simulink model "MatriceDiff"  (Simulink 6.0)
settings: Solver=ode45  StartTime=0  StopTime=17*t0  RelTol=1e-3
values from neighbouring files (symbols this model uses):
  b = S/Sm    (= 0.1)    [Constantes.m]    (also in ConstantesBck.m)
  beta = 0.95    [Constantes.m]    (also in ConstantesBck.m; ResCourV1.m = 1; ResCrV1.m = 1; ResEnerV1.m = 1)
  C = 1    [Constantes.m]    (also in ConstantesBck.m)
  gk = 36    [Constantes.m]    (also in ConstantesBck.m; sim_hh.m)
  gl = 0.3    [Constantes.m]    (also in ConstantesBck.m; sim_hh.m)
  gna = 120    [Constantes.m]    (also in ConstantesBck.m; sim_hh.m)
  h0 = 0.5961    [Constantes.m]    (also in ConstantesBck.m)
  m0 = 0.0529    [Constantes.m]    (also in ConstantesBck.m)
  mK = 0    [Constantes.m]    (also in ConstantesBck.m)
  mL = 0    [Constantes.m]    (also in ConstantesBck.m)
  mNa = 0    [Constantes.m]    (also in ConstantesBck.m)
  N = [6,8,5,5,7,1,2,6,9,1,1,9,4,8,8,7]    [Constantes.m]    (also in ConstantesBck.m; ImpedanceZtissus.m = 100; Ztissus.m = 100; charge.m = N(:,2))
  n0 = 0.3177    [Constantes.m]    (also in ConstantesBck.m)
  rapportIE = 10    [Constantes.m]
  Sm = 3.14e-2    (= 0.0314)    [Constantes.m]    (also in ConstantesBck.m = 0.000314)
  t0 = 2E-3    (= 0.002)    [Constantes.m]    (also in ConstantesBck.m = 0.001)
  Vk = -82    [Constantes.m]    (also in ConstantesBck.m)
  Vl = -59    [Constantes.m]    (also in ConstantesBck.m)
  Vna = 45    [Constantes.m]    (also in ConstantesBck.m)
  Vr = -70    [Constantes.m]    (also in ConstantesBck.m)
undefined symbols (not defined in the file or in its folder): ln
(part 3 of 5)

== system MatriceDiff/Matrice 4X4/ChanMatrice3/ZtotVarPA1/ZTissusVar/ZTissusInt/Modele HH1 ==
  HHin : Inport  Port=1  LatchInput=off
  VRefIn : Inport  Port=2  LatchInput=off
  FK : Subsystem
  FL : Fcn  Expr=gl*(u-Vl)
  FNa : Subsystem
  Gain : Gain  Gain=(1-b)/C
  Gain1 : Gain  Gain=1/(Sm*(1-b))
  Gain2 : Gain  Gain=1+mK*(b/(1-b))
  Gain3 : Gain  Gain=1+mL*(b/(1-b))
  Gain4 : Gain  Gain=1+mNa*(b/(1-b))
  Integrator : Integrator  InitialCondition=Vr
  Sum : Sum  Inputs=|---+
  Sum1 : Sum  Inputs=|++
  HHout : Outport
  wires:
  Sum/1 -> Gain/1
  Gain/1 -> Integrator/1
  FK/1(FKout) -> Gain4/1
  FNa/1(FNaOut) -> Gain2/1
  FL/1 -> Gain3/1
  HHin/1 -> Gain1/1
  Integrator/1 -> Sum1/1
  Sum1/1 -> HHout/1, FNa/1(FNaIn), FL/1, FK/1(FKIn)
  VRefIn/1 -> Sum1/2
  Gain1/1 -> Sum/4
  Gain4/1 -> Sum/1
  Gain2/1 -> Sum/2
  Gain3/1 -> Sum/3

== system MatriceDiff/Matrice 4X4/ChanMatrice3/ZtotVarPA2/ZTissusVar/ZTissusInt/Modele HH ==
  HHin : Inport  Port=1  LatchInput=off
  VRefIn : Inport  Port=2  LatchInput=off
  FK : Subsystem
  FL : Fcn  Expr=gl*(u-Vl)
  FNa : Subsystem
  Gain : Gain  Gain=(1-b)/C
  Gain1 : Gain  Gain=1/(Sm*(1-b))
  Gain2 : Gain  Gain=1+mK*(b/(1-b))
  Gain3 : Gain  Gain=1+mL*(b/(1-b))
  Gain4 : Gain  Gain=1+mNa*(b/(1-b))
  Integrator : Integrator  InitialCondition=Vr
  Sum : Sum  Inputs=|---+
  Sum1 : Sum  Inputs=|+-
  HHout : Outport
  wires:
  Sum/1 -> Gain/1
  Gain/1 -> Integrator/1
  FK/1(FKout) -> Gain4/1
  FNa/1(FNaOut) -> Gain2/1
  FL/1 -> Gain3/1
  HHin/1 -> Gain1/1
  Integrator/1 -> Sum1/1
  Sum1/1 -> HHout/1, FNa/1(FNaIn), FL/1, FK/1(FKIn)
  VRefIn/1 -> Sum1/2
  Gain1/1 -> Sum/4
  Gain4/1 -> Sum/1
  Gain2/1 -> Sum/2
  Gain3/1 -> Sum/3

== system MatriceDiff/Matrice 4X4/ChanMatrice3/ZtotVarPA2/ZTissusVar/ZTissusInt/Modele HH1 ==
  HHin : Inport  Port=1  LatchInput=off
  VRefIn : Inport  Port=2  LatchInput=off
  FK : Subsystem
  FL : Fcn  Expr=gl*(u-Vl)
  FNa : Subsystem
  Gain : Gain  Gain=(1-b)/C
  Gain1 : Gain  Gain=1/(Sm*(1-b))
  Gain2 : Gain  Gain=1+mK*(b/(1-b))
  Gain3 : Gain  Gain=1+mL*(b/(1-b))
  Gain4 : Gain  Gain=1+mNa*(b/(1-b))
  Integrator : Integrator  InitialCondition=Vr
  Sum : Sum  Inputs=|---+
  Sum1 : Sum  Inputs=|++
  HHout : Outport
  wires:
  Sum/1 -> Gain/1
  Gain/1 -> Integrator/1
  FK/1(FKout) -> Gain4/1
  FNa/1(FNaOut) -> Gain2/1
  FL/1 -> Gain3/1
  HHin/1 -> Gain1/1
  Integrator/1 -> Sum1/1
  Sum1/1 -> HHout/1, FNa/1(FNaIn), FL/1, FK/1(FKIn)
  VRefIn/1 -> Sum1/2
  Gain1/1 -> Sum/4
  Gain4/1 -> Sum/1
  Gain2/1 -> Sum/2
  Gain3/1 -> Sum/3

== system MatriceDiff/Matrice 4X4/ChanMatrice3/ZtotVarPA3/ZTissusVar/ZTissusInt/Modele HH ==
  HHin : Inport  Port=1  LatchInput=off
  VRefIn : Inport  Port=2  LatchInput=off
  FK : Subsystem
  FL : Fcn  Expr=gl*(u-Vl)
  FNa : Subsystem
  Gain : Gain  Gain=(1-b)/C
  Gain1 : Gain  Gain=1/(Sm*(1-b))
  Gain2 : Gain  Gain=1+mK*(b/(1-b))
  Gain3 : Gain  Gain=1+mL*(b/(1-b))
  Gain4 : Gain  Gain=1+mNa*(b/(1-b))
  Integrator : Integrator  InitialCondition=Vr
  Sum : Sum  Inputs=|---+
  Sum1 : Sum  Inputs=|+-
  HHout : Outport
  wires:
  Sum/1 -> Gain/1
  Gain/1 -> Integrator/1
  FK/1(FKout) -> Gain4/1
  FNa/1(FNaOut) -> Gain2/1
  FL/1 -> Gain3/1
  HHin/1 -> Gain1/1
  Integrator/1 -> Sum1/1
  Sum1/1 -> HHout/1, FNa/1(FNaIn), FL/1, FK/1(FKIn)
  VRefIn/1 -> Sum1/2
  Gain1/1 -> Sum/4
  Gain4/1 -> Sum/1
  Gain2/1 -> Sum/2
  Gain3/1 -> Sum/3

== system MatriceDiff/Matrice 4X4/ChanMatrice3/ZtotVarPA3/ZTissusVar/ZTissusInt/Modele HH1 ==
  HHin : Inport  Port=1  LatchInput=off
  VRefIn : Inport  Port=2  LatchInput=off
  FK : Subsystem
  FL : Fcn  Expr=gl*(u-Vl)
  FNa : Subsystem
  Gain : Gain  Gain=(1-b)/C
  Gain1 : Gain  Gain=1/(Sm*(1-b))
  Gain2 : Gain  Gain=1+mK*(b/(1-b))
  Gain3 : Gain  Gain=1+mL*(b/(1-b))
  Gain4 : Gain  Gain=1+mNa*(b/(1-b))
  Integrator : Integrator  InitialCondition=Vr
  Sum : Sum  Inputs=|---+
  Sum1 : Sum  Inputs=|++
  HHout : Outport
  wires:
  Sum/1 -> Gain/1
  Gain/1 -> Integrator/1
  FK/1(FKout) -> Gain4/1
  FNa/1(FNaOut) -> Gain2/1
  FL/1 -> Gain3/1
  HHin/1 -> Gain1/1
  Integrator/1 -> Sum1/1
  Sum1/1 -> HHout/1, FNa/1(FNaIn), FL/1, FK/1(FKIn)
  VRefIn/1 -> Sum1/2
  Gain1/1 -> Sum/4
  Gain4/1 -> Sum/1
  Gain2/1 -> Sum/2
  Gain3/1 -> Sum/3

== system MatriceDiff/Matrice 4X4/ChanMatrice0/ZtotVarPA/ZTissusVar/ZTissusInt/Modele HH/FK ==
  note: gkm
  note: (Vm-Vk0)
  FKIn : Inport  Port=1  LatchInput=off
  (Vm-Vk0) : Fcn  Expr=(u-Vk)
  Product : Product
  n(Vm) : Subsystem
  n^4 : Fcn  Expr=gk*(u^4)
  FKout : Outport  InitialOutput=0
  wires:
  n(Vm)/1(n) -> n^4/1
  (Vm-Vk0)/1 -> Product/2
  Product/1 -> FKout/1
  n^4/1 -> Product/1
  FKIn/1 -> n(Vm)/1(Vm), (Vm-Vk0)/1

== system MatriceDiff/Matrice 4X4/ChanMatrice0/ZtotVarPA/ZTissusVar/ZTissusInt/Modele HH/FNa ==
  note: gNa*m^3
  note: m
  note: h
  note: gNam
  note: (Vm-VNa0)
  FNaIn : Inport  Port=1  LatchInput=off
  (Vm-VNa0) : Fcn  Expr=(u-Vna)
  Product : Product
  Product1 : Product
  gna*m^3 : Fcn  Expr=gna*u^3
  h(Vm) : Subsystem
  m(Vm) : Subsystem
  FNaOut : Outport  InitialOutput=0
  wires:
  (Vm-VNa0)/1 -> Product1/2
  gna*m^3/1 -> Product/1
  Product1/1 -> FNaOut/1
  FNaIn/1 -> m(Vm)/1(Vm), h(Vm)/1(Vm), (Vm-VNa0)/1
  m(Vm)/1(n) -> gna*m^3/1
  h(Vm)/1(h) -> Product/2
  Product/1 -> Product1/1

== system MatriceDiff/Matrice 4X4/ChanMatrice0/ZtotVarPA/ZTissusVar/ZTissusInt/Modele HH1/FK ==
  note: gkm
  note: (Vm-Vk0)
  FKIn : Inport  Port=1  LatchInput=off
  (Vm-Vk0) : Fcn  Expr=(u-Vk)
  Product : Product
  n(Vm) : Subsystem
  n^4 : Fcn  Expr=gk*(u^4)
  FKout : Outport  InitialOutput=0
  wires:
  n(Vm)/1(n) -> n^4/1
  (Vm-Vk0)/1 -> Product/2
  Product/1 -> FKout/1
  n^4/1 -> Product/1
  FKIn/1 -> n(Vm)/1(Vm), (Vm-Vk0)/1

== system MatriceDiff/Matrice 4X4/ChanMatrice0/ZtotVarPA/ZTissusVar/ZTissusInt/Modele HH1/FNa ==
  note: gNa*m^3
  note: m
  note: h
  note: gNam
  note: (Vm-VNa0)
  FNaIn : Inport  Port=1  LatchInput=off
  (Vm-VNa0) : Fcn  Expr=(u-Vna)
  Product : Product
  Product1 : Product
  gna*m^3 : Fcn  Expr=gna*u^3
  h(Vm) : Subsystem
  m(Vm) : Subsystem
  FNaOut : Outport  InitialOutput=0
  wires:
  (Vm-VNa0)/1 -> Product1/2
  gna*m^3/1 -> Product/1
  Product1/1 -> FNaOut/1
  FNaIn/1 -> m(Vm)/1(Vm), h(Vm)/1(Vm), (Vm-VNa0)/1
  m(Vm)/1(n) -> gna*m^3/1
  h(Vm)/1(h) -> Product/2
  Product/1 -> Product1/1

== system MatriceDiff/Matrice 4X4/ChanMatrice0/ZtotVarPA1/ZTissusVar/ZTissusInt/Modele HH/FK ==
  note: gkm
  note: (Vm-Vk0)
  FKIn : Inport  Port=1  LatchInput=off
  (Vm-Vk0) : Fcn  Expr=(u-Vk)
  Product : Product
  n(Vm) : Subsystem
  n^4 : Fcn  Expr=gk*(u^4)
  FKout : Outport  InitialOutput=0
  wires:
  n(Vm)/1(n) -> n^4/1
  (Vm-Vk0)/1 -> Product/2
  Product/1 -> FKout/1
  n^4/1 -> Product/1
  FKIn/1 -> n(Vm)/1(Vm), (Vm-Vk0)/1

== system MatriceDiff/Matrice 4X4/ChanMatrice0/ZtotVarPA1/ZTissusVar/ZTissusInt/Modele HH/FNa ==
  note: gNa*m^3
  note: m
  note: h
  note: gNam
  note: (Vm-VNa0)
  FNaIn : Inport  Port=1  LatchInput=off
  (Vm-VNa0) : Fcn  Expr=(u-Vna)
  Product : Product
  Product1 : Product
  gna*m^3 : Fcn  Expr=gna*u^3
  h(Vm) : Subsystem
  m(Vm) : Subsystem
  FNaOut : Outport  InitialOutput=0
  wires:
  (Vm-VNa0)/1 -> Product1/2
  gna*m^3/1 -> Product/1
  Product1/1 -> FNaOut/1
  FNaIn/1 -> m(Vm)/1(Vm), h(Vm)/1(Vm), (Vm-VNa0)/1
  m(Vm)/1(n) -> gna*m^3/1
  h(Vm)/1(h) -> Product/2
  Product/1 -> Product1/1

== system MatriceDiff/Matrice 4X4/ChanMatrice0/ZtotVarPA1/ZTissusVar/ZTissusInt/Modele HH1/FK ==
  note: gkm
  note: (Vm-Vk0)
  FKIn : Inport  Port=1  LatchInput=off
  (Vm-Vk0) : Fcn  Expr=(u-Vk)
  Product : Product
  n(Vm) : Subsystem
  n^4 : Fcn  Expr=gk*(u^4)
  FKout : Outport  InitialOutput=0
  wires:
  n(Vm)/1(n) -> n^4/1
  (Vm-Vk0)/1 -> Product/2
  Product/1 -> FKout/1
  n^4/1 -> Product/1
  FKIn/1 -> n(Vm)/1(Vm), (Vm-Vk0)/1

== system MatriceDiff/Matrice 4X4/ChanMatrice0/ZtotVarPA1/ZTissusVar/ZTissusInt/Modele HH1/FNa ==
  note: gNa*m^3
  note: m
  note: h
  note: gNam
  note: (Vm-VNa0)
  FNaIn : Inport  Port=1  LatchInput=off
  (Vm-VNa0) : Fcn  Expr=(u-Vna)
  Product : Product
  Product1 : Product
  gna*m^3 : Fcn  Expr=gna*u^3
  h(Vm) : Subsystem
  m(Vm) : Subsystem
  FNaOut : Outport  InitialOutput=0
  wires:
  (Vm-VNa0)/1 -> Product1/2
  gna*m^3/1 -> Product/1
  Product1/1 -> FNaOut/1
  FNaIn/1 -> m(Vm)/1(Vm), h(Vm)/1(Vm), (Vm-VNa0)/1
  m(Vm)/1(n) -> gna*m^3/1
  h(Vm)/1(h) -> Product/2
  Product/1 -> Product1/1

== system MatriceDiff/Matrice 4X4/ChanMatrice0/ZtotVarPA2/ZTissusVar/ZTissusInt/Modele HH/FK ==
  note: gkm
  note: (Vm-Vk0)
  FKIn : Inport  Port=1  LatchInput=off
  (Vm-Vk0) : Fcn  Expr=(u-Vk)
  Product : Product
  n(Vm) : Subsystem
  n^4 : Fcn  Expr=gk*(u^4)
  FKout : Outport  InitialOutput=0
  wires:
  n(Vm)/1(n) -> n^4/1
  (Vm-Vk0)/1 -> Product/2
  Product/1 -> FKout/1
  n^4/1 -> Product/1
  FKIn/1 -> n(Vm)/1(Vm), (Vm-Vk0)/1

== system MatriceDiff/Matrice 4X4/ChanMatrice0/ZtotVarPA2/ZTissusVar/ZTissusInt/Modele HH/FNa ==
  note: gNa*m^3
  note: m
  note: h
  note: gNam
  note: (Vm-VNa0)
  FNaIn : Inport  Port=1  LatchInput=off
  (Vm-VNa0) : Fcn  Expr=(u-Vna)
  Product : Product
  Product1 : Product
  gna*m^3 : Fcn  Expr=gna*u^3
  h(Vm) : Subsystem
  m(Vm) : Subsystem
  FNaOut : Outport  InitialOutput=0
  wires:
  (Vm-VNa0)/1 -> Product1/2
  gna*m^3/1 -> Product/1
  Product1/1 -> FNaOut/1
  FNaIn/1 -> m(Vm)/1(Vm), h(Vm)/1(Vm), (Vm-VNa0)/1
  m(Vm)/1(n) -> gna*m^3/1
  h(Vm)/1(h) -> Product/2
  Product/1 -> Product1/1

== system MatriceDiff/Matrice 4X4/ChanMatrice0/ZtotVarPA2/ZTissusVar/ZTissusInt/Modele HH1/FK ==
  note: gkm
  note: (Vm-Vk0)
  FKIn : Inport  Port=1  LatchInput=off
  (Vm-Vk0) : Fcn  Expr=(u-Vk)
  Product : Product
  n(Vm) : Subsystem
  n^4 : Fcn  Expr=gk*(u^4)
  FKout : Outport  InitialOutput=0
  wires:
  n(Vm)/1(n) -> n^4/1
  (Vm-Vk0)/1 -> Product/2
  Product/1 -> FKout/1
  n^4/1 -> Product/1
  FKIn/1 -> n(Vm)/1(Vm), (Vm-Vk0)/1

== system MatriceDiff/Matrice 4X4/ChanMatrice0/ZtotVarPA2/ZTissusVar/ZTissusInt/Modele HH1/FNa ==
  note: gNa*m^3
  note: m
  note: h
  note: gNam
  note: (Vm-VNa0)
  FNaIn : Inport  Port=1  LatchInput=off
  (Vm-VNa0) : Fcn  Expr=(u-Vna)
  Product : Product
  Product1 : Product
  gna*m^3 : Fcn  Expr=gna*u^3
  h(Vm) : Subsystem
  m(Vm) : Subsystem
  FNaOut : Outport  InitialOutput=0
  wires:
  (Vm-VNa0)/1 -> Product1/2
  gna*m^3/1 -> Product/1
  Product1/1 -> FNaOut/1
  FNaIn/1 -> m(Vm)/1(Vm), h(Vm)/1(Vm), (Vm-VNa0)/1
  m(Vm)/1(n) -> gna*m^3/1
  h(Vm)/1(h) -> Product/2
  Product/1 -> Product1/1

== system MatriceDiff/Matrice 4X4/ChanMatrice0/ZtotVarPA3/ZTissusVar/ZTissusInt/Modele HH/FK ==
  note: gkm
  note: (Vm-Vk0)
  FKIn : Inport  Port=1  LatchInput=off
  (Vm-Vk0) : Fcn  Expr=(u-Vk)
  Product : Product
  n(Vm) : Subsystem
  n^4 : Fcn  Expr=gk*(u^4)
  FKout : Outport  InitialOutput=0
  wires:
  n(Vm)/1(n) -> n^4/1
  (Vm-Vk0)/1 -> Product/2
  Product/1 -> FKout/1
  n^4/1 -> Product/1
  FKIn/1 -> n(Vm)/1(Vm), (Vm-Vk0)/1

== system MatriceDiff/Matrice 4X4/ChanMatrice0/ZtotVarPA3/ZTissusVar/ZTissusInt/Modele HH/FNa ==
  note: gNa*m^3
  note: m
  note: h
  note: gNam
  note: (Vm-VNa0)
  FNaIn : Inport  Port=1  LatchInput=off
  (Vm-VNa0) : Fcn  Expr=(u-Vna)
  Product : Product
  Product1 : Product
  gna*m^3 : Fcn  Expr=gna*u^3
  h(Vm) : Subsystem
  m(Vm) : Subsystem
  FNaOut : Outport  InitialOutput=0
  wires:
  (Vm-VNa0)/1 -> Product1/2
  gna*m^3/1 -> Product/1
  Product1/1 -> FNaOut/1
  FNaIn/1 -> m(Vm)/1(Vm), h(Vm)/1(Vm), (Vm-VNa0)/1
  m(Vm)/1(n) -> gna*m^3/1
  h(Vm)/1(h) -> Product/2
  Product/1 -> Product1/1

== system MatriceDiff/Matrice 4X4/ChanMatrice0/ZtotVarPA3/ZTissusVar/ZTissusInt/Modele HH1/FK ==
  note: gkm
  note: (Vm-Vk0)
  FKIn : Inport  Port=1  LatchInput=off
  (Vm-Vk0) : Fcn  Expr=(u-Vk)
  Product : Product
  n(Vm) : Subsystem
  n^4 : Fcn  Expr=gk*(u^4)
  FKout : Outport  InitialOutput=0
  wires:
  n(Vm)/1(n) -> n^4/1
  (Vm-Vk0)/1 -> Product/2
  Product/1 -> FKout/1
  n^4/1 -> Product/1
  FKIn/1 -> n(Vm)/1(Vm), (Vm-Vk0)/1

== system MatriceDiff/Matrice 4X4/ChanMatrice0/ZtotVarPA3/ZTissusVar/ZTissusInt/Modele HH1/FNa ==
  note: gNa*m^3
  note: m
  note: h
  note: gNam
  note: (Vm-VNa0)
  FNaIn : Inport  Port=1  LatchInput=off
  (Vm-VNa0) : Fcn  Expr=(u-Vna)
  Product : Product
  Product1 : Product
  gna*m^3 : Fcn  Expr=gna*u^3
  h(Vm) : Subsystem
  m(Vm) : Subsystem
  FNaOut : Outport  InitialOutput=0
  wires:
  (Vm-VNa0)/1 -> Product1/2
  gna*m^3/1 -> Product/1
  Product1/1 -> FNaOut/1
  FNaIn/1 -> m(Vm)/1(Vm), h(Vm)/1(Vm), (Vm-VNa0)/1
  m(Vm)/1(n) -> gna*m^3/1
  h(Vm)/1(h) -> Product/2
  Product/1 -> Product1/1

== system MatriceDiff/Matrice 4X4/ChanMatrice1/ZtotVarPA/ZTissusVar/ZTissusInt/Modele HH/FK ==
  note: gkm
  note: (Vm-Vk0)
  FKIn : Inport  Port=1  LatchInput=off
  (Vm-Vk0) : Fcn  Expr=(u-Vk)
  Product : Product
  n(Vm) : Subsystem
  n^4 : Fcn  Expr=gk*(u^4)
  FKout : Outport  InitialOutput=0
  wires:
  n(Vm)/1(n) -> n^4/1
  (Vm-Vk0)/1 -> Product/2
  Product/1 -> FKout/1
  n^4/1 -> Product/1
  FKIn/1 -> n(Vm)/1(Vm), (Vm-Vk0)/1

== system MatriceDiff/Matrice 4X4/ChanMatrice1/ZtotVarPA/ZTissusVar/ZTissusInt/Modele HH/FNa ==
  note: gNa*m^3
  note: m
  note: h
  note: gNam
  note: (Vm-VNa0)
  FNaIn : Inport  Port=1  LatchInput=off
  (Vm-VNa0) : Fcn  Expr=(u-Vna)
  Product : Product
  Product1 : Product
  gna*m^3 : Fcn  Expr=gna*u^3
  h(Vm) : Subsystem
  m(Vm) : Subsystem
  FNaOut : Outport  InitialOutput=0
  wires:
  (Vm-VNa0)/1 -> Product1/2
  gna*m^3/1 -> Product/1
  Product1/1 -> FNaOut/1
  FNaIn/1 -> m(Vm)/1(Vm), h(Vm)/1(Vm), (Vm-VNa0)/1
  m(Vm)/1(n) -> gna*m^3/1
  h(Vm)/1(h) -> Product/2
  Product/1 -> Product1/1

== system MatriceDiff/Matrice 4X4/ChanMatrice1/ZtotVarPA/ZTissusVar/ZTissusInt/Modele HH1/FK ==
  note: gkm
  note: (Vm-Vk0)
  FKIn : Inport  Port=1  LatchInput=off
  (Vm-Vk0) : Fcn  Expr=(u-Vk)
  Product : Product
  n(Vm) : Subsystem
  n^4 : Fcn  Expr=gk*(u^4)
  FKout : Outport  InitialOutput=0
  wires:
  n(Vm)/1(n) -> n^4/1
  (Vm-Vk0)/1 -> Product/2
  Product/1 -> FKout/1
  n^4/1 -> Product/1
  FKIn/1 -> n(Vm)/1(Vm), (Vm-Vk0)/1

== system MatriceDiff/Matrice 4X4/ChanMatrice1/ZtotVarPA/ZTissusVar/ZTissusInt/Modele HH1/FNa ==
  note: gNa*m^3
  note: m
  note: h
  note: gNam
  note: (Vm-VNa0)
  FNaIn : Inport  Port=1  LatchInput=off
  (Vm-VNa0) : Fcn  Expr=(u-Vna)
  Product : Product
  Product1 : Product
  gna*m^3 : Fcn  Expr=gna*u^3
  h(Vm) : Subsystem
  m(Vm) : Subsystem
  FNaOut : Outport  InitialOutput=0
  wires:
  (Vm-VNa0)/1 -> Product1/2
  gna*m^3/1 -> Product/1
  Product1/1 -> FNaOut/1
  FNaIn/1 -> m(Vm)/1(Vm), h(Vm)/1(Vm), (Vm-VNa0)/1
  m(Vm)/1(n) -> gna*m^3/1
  h(Vm)/1(h) -> Product/2
  Product/1 -> Product1/1

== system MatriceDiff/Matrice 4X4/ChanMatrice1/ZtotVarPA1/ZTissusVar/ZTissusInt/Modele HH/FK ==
  note: gkm
  note: (Vm-Vk0)
  FKIn : Inport  Port=1  LatchInput=off
  (Vm-Vk0) : Fcn  Expr=(u-Vk)
  Product : Product
  n(Vm) : Subsystem
  n^4 : Fcn  Expr=gk*(u^4)
  FKout : Outport  InitialOutput=0
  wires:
  n(Vm)/1(n) -> n^4/1
  (Vm-Vk0)/1 -> Product/2
  Product/1 -> FKout/1
  n^4/1 -> Product/1
  FKIn/1 -> n(Vm)/1(Vm), (Vm-Vk0)/1

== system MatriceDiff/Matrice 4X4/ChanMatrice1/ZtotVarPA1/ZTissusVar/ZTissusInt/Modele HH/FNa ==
  note: gNa*m^3
  note: m
  note: h
  note: gNam
  note: (Vm-VNa0)
  FNaIn : Inport  Port=1  LatchInput=off
  (Vm-VNa0) : Fcn  Expr=(u-Vna)
  Product : Product
  Product1 : Product
  gna*m^3 : Fcn  Expr=gna*u^3
  h(Vm) : Subsystem
  m(Vm) : Subsystem
  FNaOut : Outport  InitialOutput=0
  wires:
  (Vm-VNa0)/1 -> Product1/2
  gna*m^3/1 -> Product/1
  Product1/1 -> FNaOut/1
  FNaIn/1 -> m(Vm)/1(Vm), h(Vm)/1(Vm), (Vm-VNa0)/1
  m(Vm)/1(n) -> gna*m^3/1
  h(Vm)/1(h) -> Product/2
  Product/1 -> Product1/1

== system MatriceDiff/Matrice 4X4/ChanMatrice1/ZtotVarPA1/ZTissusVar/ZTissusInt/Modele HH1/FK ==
  note: gkm
  note: (Vm-Vk0)
  FKIn : Inport  Port=1  LatchInput=off
  (Vm-Vk0) : Fcn  Expr=(u-Vk)
  Product : Product
  n(Vm) : Subsystem
  n^4 : Fcn  Expr=gk*(u^4)
  FKout : Outport  InitialOutput=0
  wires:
  n(Vm)/1(n) -> n^4/1
  (Vm-Vk0)/1 -> Product/2
  Product/1 -> FKout/1
  n^4/1 -> Product/1
  FKIn/1 -> n(Vm)/1(Vm), (Vm-Vk0)/1

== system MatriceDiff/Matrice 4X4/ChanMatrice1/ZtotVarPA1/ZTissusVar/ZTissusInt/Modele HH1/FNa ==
  note: gNa*m^3
  note: m
  note: h
  note: gNam
  note: (Vm-VNa0)
  FNaIn : Inport  Port=1  LatchInput=off
  (Vm-VNa0) : Fcn  Expr=(u-Vna)
  Product : Product
  Product1 : Product
  gna*m^3 : Fcn  Expr=gna*u^3
  h(Vm) : Subsystem
  m(Vm) : Subsystem
  FNaOut : Outport  InitialOutput=0
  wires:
  (Vm-VNa0)/1 -> Product1/2
  gna*m^3/1 -> Product/1
  Product1/1 -> FNaOut/1
  FNaIn/1 -> m(Vm)/1(Vm), h(Vm)/1(Vm), (Vm-VNa0)/1
  m(Vm)/1(n) -> gna*m^3/1
  h(Vm)/1(h) -> Product/2
  Product/1 -> Product1/1

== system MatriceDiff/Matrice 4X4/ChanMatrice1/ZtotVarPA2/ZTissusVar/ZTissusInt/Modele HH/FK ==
  note: gkm
  note: (Vm-Vk0)
  FKIn : Inport  Port=1  LatchInput=off
  (Vm-Vk0) : Fcn  Expr=(u-Vk)
  Product : Product
  n(Vm) : Subsystem
  n^4 : Fcn  Expr=gk*(u^4)
  FKout : Outport  InitialOutput=0
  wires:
  n(Vm)/1(n) -> n^4/1
  (Vm-Vk0)/1 -> Product/2
  Product/1 -> FKout/1
  n^4/1 -> Product/1
  FKIn/1 -> n(Vm)/1(Vm), (Vm-Vk0)/1

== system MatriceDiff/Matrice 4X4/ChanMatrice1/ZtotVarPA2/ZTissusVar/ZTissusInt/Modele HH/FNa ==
  note: gNa*m^3
  note: m
  note: h
  note: gNam
  note: (Vm-VNa0)
  FNaIn : Inport  Port=1  LatchInput=off
  (Vm-VNa0) : Fcn  Expr=(u-Vna)
  Product : Product
  Product1 : Product
  gna*m^3 : Fcn  Expr=gna*u^3
  h(Vm) : Subsystem
  m(Vm) : Subsystem
  FNaOut : Outport  InitialOutput=0
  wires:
  (Vm-VNa0)/1 -> Product1/2
  gna*m^3/1 -> Product/1
  Product1/1 -> FNaOut/1
  FNaIn/1 -> m(Vm)/1(Vm), h(Vm)/1(Vm), (Vm-VNa0)/1
  m(Vm)/1(n) -> gna*m^3/1
  h(Vm)/1(h) -> Product/2
  Product/1 -> Product1/1

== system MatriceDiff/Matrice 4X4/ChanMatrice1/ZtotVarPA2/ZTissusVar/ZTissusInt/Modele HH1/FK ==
  note: gkm
  note: (Vm-Vk0)
  FKIn : Inport  Port=1  LatchInput=off
  (Vm-Vk0) : Fcn  Expr=(u-Vk)
  Product : Product
  n(Vm) : Subsystem
  n^4 : Fcn  Expr=gk*(u^4)
  FKout : Outport  InitialOutput=0
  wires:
  n(Vm)/1(n) -> n^4/1
  (Vm-Vk0)/1 -> Product/2
  Product/1 -> FKout/1
  n^4/1 -> Product/1
  FKIn/1 -> n(Vm)/1(Vm), (Vm-Vk0)/1

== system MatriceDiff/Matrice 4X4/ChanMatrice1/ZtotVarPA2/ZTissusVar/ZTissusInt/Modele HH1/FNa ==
  note: gNa*m^3
  note: m
  note: h
  note: gNam
  note: (Vm-VNa0)
  FNaIn : Inport  Port=1  LatchInput=off
  (Vm-VNa0) : Fcn  Expr=(u-Vna)
  Product : Product
  Product1 : Product
  gna*m^3 : Fcn  Expr=gna*u^3
  h(Vm) : Subsystem
  m(Vm) : Subsystem
  FNaOut : Outport  InitialOutput=0
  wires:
  (Vm-VNa0)/1 -> Product1/2
  gna*m^3/1 -> Product/1
  Product1/1 -> FNaOut/1
  FNaIn/1 -> m(Vm)/1(Vm), h(Vm)/1(Vm), (Vm-VNa0)/1
  m(Vm)/1(n) -> gna*m^3/1
  h(Vm)/1(h) -> Product/2
  Product/1 -> Product1/1

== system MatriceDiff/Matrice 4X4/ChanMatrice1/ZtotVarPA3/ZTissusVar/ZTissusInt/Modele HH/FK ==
  note: gkm
  note: (Vm-Vk0)
  FKIn : Inport  Port=1  LatchInput=off
  (Vm-Vk0) : Fcn  Expr=(u-Vk)
  Product : Product
  n(Vm) : Subsystem
  n^4 : Fcn  Expr=gk*(u^4)
  FKout : Outport  InitialOutput=0
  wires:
  n(Vm)/1(n) -> n^4/1
  (Vm-Vk0)/1 -> Product/2
  Product/1 -> FKout/1
  n^4/1 -> Product/1
  FKIn/1 -> n(Vm)/1(Vm), (Vm-Vk0)/1

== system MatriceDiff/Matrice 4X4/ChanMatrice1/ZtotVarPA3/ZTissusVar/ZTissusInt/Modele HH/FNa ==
  note: gNa*m^3
  note: m
  note: h
  note: gNam
  note: (Vm-VNa0)
  FNaIn : Inport  Port=1  LatchInput=off
  (Vm-VNa0) : Fcn  Expr=(u-Vna)
  Product : Product
  Product1 : Product
  gna*m^3 : Fcn  Expr=gna*u^3
  h(Vm) : Subsystem
  m(Vm) : Subsystem
  FNaOut : Outport  InitialOutput=0
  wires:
  (Vm-VNa0)/1 -> Product1/2
  gna*m^3/1 -> Product/1
  Product1/1 -> FNaOut/1
  FNaIn/1 -> m(Vm)/1(Vm), h(Vm)/1(Vm), (Vm-VNa0)/1
  m(Vm)/1(n) -> gna*m^3/1
  h(Vm)/1(h) -> Product/2
  Product/1 -> Product1/1

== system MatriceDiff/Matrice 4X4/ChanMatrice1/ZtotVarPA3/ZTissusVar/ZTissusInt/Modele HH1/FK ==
  note: gkm
  note: (Vm-Vk0)
  FKIn : Inport  Port=1  LatchInput=off
  (Vm-Vk0) : Fcn  Expr=(u-Vk)
  Product : Product
  n(Vm) : Subsystem
  n^4 : Fcn  Expr=gk*(u^4)
  FKout : Outport  InitialOutput=0
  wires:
  n(Vm)/1(n) -> n^4/1
  (Vm-Vk0)/1 -> Product/2
  Product/1 -> FKout/1
  n^4/1 -> Product/1
  FKIn/1 -> n(Vm)/1(Vm), (Vm-Vk0)/1

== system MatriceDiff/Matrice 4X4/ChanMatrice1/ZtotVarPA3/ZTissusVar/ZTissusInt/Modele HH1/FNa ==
  note: gNa*m^3
  note: m
  note: h
  note: gNam
  note: (Vm-VNa0)
  FNaIn : Inport  Port=1  LatchInput=off
  (Vm-VNa0) : Fcn  Expr=(u-Vna)
  Product : Product
  Product1 : Product
  gna*m^3 : Fcn  Expr=gna*u^3
  h(Vm) : Subsystem
  m(Vm) : Subsystem
  FNaOut : Outport  InitialOutput=0
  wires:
  (Vm-VNa0)/1 -> Product1/2
  gna*m^3/1 -> Product/1
  Product1/1 -> FNaOut/1
  FNaIn/1 -> m(Vm)/1(Vm), h(Vm)/1(Vm), (Vm-VNa0)/1
  m(Vm)/1(n) -> gna*m^3/1
  h(Vm)/1(h) -> Product/2
  Product/1 -> Product1/1

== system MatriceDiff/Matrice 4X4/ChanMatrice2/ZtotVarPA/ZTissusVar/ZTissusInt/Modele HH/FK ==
  note: gkm
  note: (Vm-Vk0)
  FKIn : Inport  Port=1  LatchInput=off
  (Vm-Vk0) : Fcn  Expr=(u-Vk)
  Product : Product
  n(Vm) : Subsystem
  n^4 : Fcn  Expr=gk*(u^4)
  FKout : Outport  InitialOutput=0
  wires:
  n(Vm)/1(n) -> n^4/1
  (Vm-Vk0)/1 -> Product/2
  Product/1 -> FKout/1
  n^4/1 -> Product/1
  FKIn/1 -> n(Vm)/1(Vm), (Vm-Vk0)/1

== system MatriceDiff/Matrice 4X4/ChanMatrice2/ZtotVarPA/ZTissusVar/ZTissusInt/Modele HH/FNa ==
  note: gNa*m^3
  note: m
  note: h
  note: gNam
  note: (Vm-VNa0)
  FNaIn : Inport  Port=1  LatchInput=off
  (Vm-VNa0) : Fcn  Expr=(u-Vna)
  Product : Product
  Product1 : Product
  gna*m^3 : Fcn  Expr=gna*u^3
  h(Vm) : Subsystem
  m(Vm) : Subsystem
  FNaOut : Outport  InitialOutput=0
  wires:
  (Vm-VNa0)/1 -> Product1/2
  gna*m^3/1 -> Product/1
  Product1/1 -> FNaOut/1
  FNaIn/1 -> m(Vm)/1(Vm), h(Vm)/1(Vm), (Vm-VNa0)/1
  m(Vm)/1(n) -> gna*m^3/1
  h(Vm)/1(h) -> Product/2
  Product/1 -> Product1/1

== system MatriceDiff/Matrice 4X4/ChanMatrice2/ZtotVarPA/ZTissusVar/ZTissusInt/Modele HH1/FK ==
  note: gkm
  note: (Vm-Vk0)
  FKIn : Inport  Port=1  LatchInput=off
  (Vm-Vk0) : Fcn  Expr=(u-Vk)
  Product : Product
  n(Vm) : Subsystem
  n^4 : Fcn  Expr=gk*(u^4)
  FKout : Outport  InitialOutput=0
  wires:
  n(Vm)/1(n) -> n^4/1
  (Vm-Vk0)/1 -> Product/2
  Product/1 -> FKout/1
  n^4/1 -> Product/1
  FKIn/1 -> n(Vm)/1(Vm), (Vm-Vk0)/1

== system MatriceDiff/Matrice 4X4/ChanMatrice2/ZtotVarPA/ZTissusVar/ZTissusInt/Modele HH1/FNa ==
  note: gNa*m^3
  note: m
  note: h
  note: gNam
  note: (Vm-VNa0)
  FNaIn : Inport  Port=1  LatchInput=off
  (Vm-VNa0) : Fcn  Expr=(u-Vna)
  Product : Product
  Product1 : Product
  gna*m^3 : Fcn  Expr=gna*u^3
  h(Vm) : Subsystem
  m(Vm) : Subsystem
  FNaOut : Outport  InitialOutput=0
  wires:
  (Vm-VNa0)/1 -> Product1/2
  gna*m^3/1 -> Product/1
  Product1/1 -> FNaOut/1
  FNaIn/1 -> m(Vm)/1(Vm), h(Vm)/1(Vm), (Vm-VNa0)/1
  m(Vm)/1(n) -> gna*m^3/1
  h(Vm)/1(h) -> Product/2
  Product/1 -> Product1/1

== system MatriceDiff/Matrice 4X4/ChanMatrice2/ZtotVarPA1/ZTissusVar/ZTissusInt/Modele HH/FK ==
  note: gkm
  note: (Vm-Vk0)
  FKIn : Inport  Port=1  LatchInput=off
  (Vm-Vk0) : Fcn  Expr=(u-Vk)
  Product : Product
  n(Vm) : Subsystem
  n^4 : Fcn  Expr=gk*(u^4)
  FKout : Outport  InitialOutput=0
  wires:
  n(Vm)/1(n) -> n^4/1
  (Vm-Vk0)/1 -> Product/2
  Product/1 -> FKout/1
  n^4/1 -> Product/1
  FKIn/1 -> n(Vm)/1(Vm), (Vm-Vk0)/1

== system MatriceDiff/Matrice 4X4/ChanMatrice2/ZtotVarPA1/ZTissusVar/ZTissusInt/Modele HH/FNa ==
  note: gNa*m^3
  note: m
  note: h
  note: gNam
  note: (Vm-VNa0)
  FNaIn : Inport  Port=1  LatchInput=off
  (Vm-VNa0) : Fcn  Expr=(u-Vna)
  Product : Product
  Product1 : Product
  gna*m^3 : Fcn  Expr=gna*u^3
  h(Vm) : Subsystem
  m(Vm) : Subsystem
  FNaOut : Outport  InitialOutput=0
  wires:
  (Vm-VNa0)/1 -> Product1/2
  gna*m^3/1 -> Product/1
  Product1/1 -> FNaOut/1
  FNaIn/1 -> m(Vm)/1(Vm), h(Vm)/1(Vm), (Vm-VNa0)/1
  m(Vm)/1(n) -> gna*m^3/1
  h(Vm)/1(h) -> Product/2
  Product/1 -> Product1/1

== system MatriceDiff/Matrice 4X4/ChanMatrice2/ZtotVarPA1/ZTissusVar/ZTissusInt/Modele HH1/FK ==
  note: gkm
  note: (Vm-Vk0)
  FKIn : Inport  Port=1  LatchInput=off
  (Vm-Vk0) : Fcn  Expr=(u-Vk)
  Product : Product
  n(Vm) : Subsystem
  n^4 : Fcn  Expr=gk*(u^4)
  FKout : Outport  InitialOutput=0
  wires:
  n(Vm)/1(n) -> n^4/1
  (Vm-Vk0)/1 -> Product/2
  Product/1 -> FKout/1
  n^4/1 -> Product/1
  FKIn/1 -> n(Vm)/1(Vm), (Vm-Vk0)/1

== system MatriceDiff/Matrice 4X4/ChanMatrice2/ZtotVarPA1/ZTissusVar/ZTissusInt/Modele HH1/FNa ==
  note: gNa*m^3
  note: m
  note: h
  note: gNam
  note: (Vm-VNa0)
  FNaIn : Inport  Port=1  LatchInput=off
  (Vm-VNa0) : Fcn  Expr=(u-Vna)
  Product : Product
  Product1 : Product
  gna*m^3 : Fcn  Expr=gna*u^3
  h(Vm) : Subsystem
  m(Vm) : Subsystem
  FNaOut : Outport  InitialOutput=0
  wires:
  (Vm-VNa0)/1 -> Product1/2
  gna*m^3/1 -> Product/1
  Product1/1 -> FNaOut/1
  FNaIn/1 -> m(Vm)/1(Vm), h(Vm)/1(Vm), (Vm-VNa0)/1
  m(Vm)/1(n) -> gna*m^3/1
  h(Vm)/1(h) -> Product/2
  Product/1 -> Product1/1

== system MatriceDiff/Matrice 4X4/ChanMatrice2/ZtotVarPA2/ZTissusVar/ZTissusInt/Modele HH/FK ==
  note: gkm
  note: (Vm-Vk0)
  FKIn : Inport  Port=1  LatchInput=off
  (Vm-Vk0) : Fcn  Expr=(u-Vk)
  Product : Product
  n(Vm) : Subsystem
  n^4 : Fcn  Expr=gk*(u^4)
  FKout : Outport  InitialOutput=0
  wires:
  n(Vm)/1(n) -> n^4/1
  (Vm-Vk0)/1 -> Product/2
  Product/1 -> FKout/1
  n^4/1 -> Product/1
  FKIn/1 -> n(Vm)/1(Vm), (Vm-Vk0)/1

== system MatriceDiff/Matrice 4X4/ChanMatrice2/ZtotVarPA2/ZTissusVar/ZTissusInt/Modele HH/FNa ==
  note: gNa*m^3
  note: m
  note: h
  note: gNam
  note: (Vm-VNa0)
  FNaIn : Inport  Port=1  LatchInput=off
  (Vm-VNa0) : Fcn  Expr=(u-Vna)
  Product : Product
  Product1 : Product
  gna*m^3 : Fcn  Expr=gna*u^3
  h(Vm) : Subsystem
  m(Vm) : Subsystem
  FNaOut : Outport  InitialOutput=0
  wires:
  (Vm-VNa0)/1 -> Product1/2
  gna*m^3/1 -> Product/1
  Product1/1 -> FNaOut/1
  FNaIn/1 -> m(Vm)/1(Vm), h(Vm)/1(Vm), (Vm-VNa0)/1
  m(Vm)/1(n) -> gna*m^3/1
  h(Vm)/1(h) -> Product/2
  Product/1 -> Product1/1

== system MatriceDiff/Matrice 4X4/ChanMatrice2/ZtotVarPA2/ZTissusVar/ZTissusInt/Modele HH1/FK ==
  note: gkm
  note: (Vm-Vk0)
  FKIn : Inport  Port=1  LatchInput=off
  (Vm-Vk0) : Fcn  Expr=(u-Vk)
  Product : Product
  n(Vm) : Subsystem
  n^4 : Fcn  Expr=gk*(u^4)
  FKout : Outport  InitialOutput=0
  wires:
  n(Vm)/1(n) -> n^4/1
  (Vm-Vk0)/1 -> Product/2
  Product/1 -> FKout/1
  n^4/1 -> Product/1
  FKIn/1 -> n(Vm)/1(Vm), (Vm-Vk0)/1

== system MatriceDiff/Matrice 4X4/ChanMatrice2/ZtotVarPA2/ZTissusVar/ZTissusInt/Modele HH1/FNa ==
  note: gNa*m^3
  note: m
  note: h
  note: gNam
  note: (Vm-VNa0)
  FNaIn : Inport  Port=1  LatchInput=off
  (Vm-VNa0) : Fcn  Expr=(u-Vna)
  Product : Product
  Product1 : Product
  gna*m^3 : Fcn  Expr=gna*u^3
  h(Vm) : Subsystem
  m(Vm) : Subsystem
  FNaOut : Outport  InitialOutput=0
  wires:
  (Vm-VNa0)/1 -> Product1/2
  gna*m^3/1 -> Product/1
  Product1/1 -> FNaOut/1
  FNaIn/1 -> m(Vm)/1(Vm), h(Vm)/1(Vm), (Vm-VNa0)/1
  m(Vm)/1(n) -> gna*m^3/1
  h(Vm)/1(h) -> Product/2
  Product/1 -> Product1/1

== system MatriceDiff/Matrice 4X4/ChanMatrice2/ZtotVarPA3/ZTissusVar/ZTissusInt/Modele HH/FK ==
  note: gkm
  note: (Vm-Vk0)
  FKIn : Inport  Port=1  LatchInput=off
  (Vm-Vk0) : Fcn  Expr=(u-Vk)
  Product : Product
  n(Vm) : Subsystem
  n^4 : Fcn  Expr=gk*(u^4)
  FKout : Outport  InitialOutput=0
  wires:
  n(Vm)/1(n) -> n^4/1
  (Vm-Vk0)/1 -> Product/2
  Product/1 -> FKout/1
  n^4/1 -> Product/1
  FKIn/1 -> n(Vm)/1(Vm), (Vm-Vk0)/1

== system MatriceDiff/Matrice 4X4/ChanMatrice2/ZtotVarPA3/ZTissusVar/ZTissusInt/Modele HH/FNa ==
  note: gNa*m^3
  note: m
  note: h
  note: gNam
  note: (Vm-VNa0)
  FNaIn : Inport  Port=1  LatchInput=off
  (Vm-VNa0) : Fcn  Expr=(u-Vna)
  Product : Product
  Product1 : Product
  gna*m^3 : Fcn  Expr=gna*u^3
  h(Vm) : Subsystem
  m(Vm) : Subsystem
  FNaOut : Outport  InitialOutput=0
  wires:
  (Vm-VNa0)/1 -> Product1/2
  gna*m^3/1 -> Product/1
  Product1/1 -> FNaOut/1
  FNaIn/1 -> m(Vm)/1(Vm), h(Vm)/1(Vm), (Vm-VNa0)/1
  m(Vm)/1(n) -> gna*m^3/1
  h(Vm)/1(h) -> Product/2
  Product/1 -> Product1/1

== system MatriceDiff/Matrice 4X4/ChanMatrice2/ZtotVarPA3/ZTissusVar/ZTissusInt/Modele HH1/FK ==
  note: gkm
  note: (Vm-Vk0)
  FKIn : Inport  Port=1  LatchInput=off
  (Vm-Vk0) : Fcn  Expr=(u-Vk)
  Product : Product
  n(Vm) : Subsystem
  n^4 : Fcn  Expr=gk*(u^4)
  FKout : Outport  InitialOutput=0
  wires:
  n(Vm)/1(n) -> n^4/1
  (Vm-Vk0)/1 -> Product/2
  Product/1 -> FKout/1
  n^4/1 -> Product/1
  FKIn/1 -> n(Vm)/1(Vm), (Vm-Vk0)/1

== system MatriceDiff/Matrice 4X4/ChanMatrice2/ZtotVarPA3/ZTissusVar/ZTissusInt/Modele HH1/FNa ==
  note: gNa*m^3
  note: m
  note: h
  note: gNam
  note: (Vm-VNa0)
  FNaIn : Inport  Port=1  LatchInput=off
  (Vm-VNa0) : Fcn  Expr=(u-Vna)
  Product : Product
  Product1 : Product
  gna*m^3 : Fcn  Expr=gna*u^3
  h(Vm) : Subsystem
  m(Vm) : Subsystem
  FNaOut : Outport  InitialOutput=0
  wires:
  (Vm-VNa0)/1 -> Product1/2
  gna*m^3/1 -> Product/1
  Product1/1 -> FNaOut/1
  FNaIn/1 -> m(Vm)/1(Vm), h(Vm)/1(Vm), (Vm-VNa0)/1
  m(Vm)/1(n) -> gna*m^3/1
  h(Vm)/1(h) -> Product/2
  Product/1 -> Product1/1

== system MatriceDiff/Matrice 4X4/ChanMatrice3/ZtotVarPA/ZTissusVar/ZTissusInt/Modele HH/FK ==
  note: gkm
  note: (Vm-Vk0)
  FKIn : Inport  Port=1  LatchInput=off
  (Vm-Vk0) : Fcn  Expr=(u-Vk)
  Product : Product
  n(Vm) : Subsystem
  n^4 : Fcn  Expr=gk*(u^4)
  FKout : Outport  InitialOutput=0
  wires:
  n(Vm)/1(n) -> n^4/1
  (Vm-Vk0)/1 -> Product/2
  Product/1 -> FKout/1
  n^4/1 -> Product/1
  FKIn/1 -> n(Vm)/1(Vm), (Vm-Vk0)/1

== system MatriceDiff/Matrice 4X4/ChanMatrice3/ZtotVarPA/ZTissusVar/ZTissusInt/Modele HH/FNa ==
  note: gNa*m^3
  note: m
  note: h
  note: gNam
  note: (Vm-VNa0)
  FNaIn : Inport  Port=1  LatchInput=off
  (Vm-VNa0) : Fcn  Expr=(u-Vna)
  Product : Product
  Product1 : Product
  gna*m^3 : Fcn  Expr=gna*u^3
  h(Vm) : Subsystem
  m(Vm) : Subsystem
  FNaOut : Outport  InitialOutput=0
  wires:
  (Vm-VNa0)/1 -> Product1/2
  gna*m^3/1 -> Product/1
  Product1/1 -> FNaOut/1
  FNaIn/1 -> m(Vm)/1(Vm), h(Vm)/1(Vm), (Vm-VNa0)/1
  m(Vm)/1(n) -> gna*m^3/1
  h(Vm)/1(h) -> Product/2
  Product/1 -> Product1/1

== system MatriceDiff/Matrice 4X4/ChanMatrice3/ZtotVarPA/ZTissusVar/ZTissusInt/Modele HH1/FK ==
  note: gkm
  note: (Vm-Vk0)
  FKIn : Inport  Port=1  LatchInput=off
  (Vm-Vk0) : Fcn  Expr=(u-Vk)
  Product : Product
  n(Vm) : Subsystem
  n^4 : Fcn  Expr=gk*(u^4)
  FKout : Outport  InitialOutput=0
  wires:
  n(Vm)/1(n) -> n^4/1
  (Vm-Vk0)/1 -> Product/2
  Product/1 -> FKout/1
  n^4/1 -> Product/1
  FKIn/1 -> n(Vm)/1(Vm), (Vm-Vk0)/1

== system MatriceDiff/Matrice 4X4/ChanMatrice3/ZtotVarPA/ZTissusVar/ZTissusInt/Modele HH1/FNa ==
  note: gNa*m^3
  note: m
  note: h
  note: gNam
  note: (Vm-VNa0)
  FNaIn : Inport  Port=1  LatchInput=off
  (Vm-VNa0) : Fcn  Expr=(u-Vna)
  Product : Product
  Product1 : Product
  gna*m^3 : Fcn  Expr=gna*u^3
  h(Vm) : Subsystem
  m(Vm) : Subsystem
  FNaOut : Outport  InitialOutput=0
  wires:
  (Vm-VNa0)/1 -> Product1/2
  gna*m^3/1 -> Product/1
  Product1/1 -> FNaOut/1
  FNaIn/1 -> m(Vm)/1(Vm), h(Vm)/1(Vm), (Vm-VNa0)/1
  m(Vm)/1(n) -> gna*m^3/1
  h(Vm)/1(h) -> Product/2
  Product/1 -> Product1/1

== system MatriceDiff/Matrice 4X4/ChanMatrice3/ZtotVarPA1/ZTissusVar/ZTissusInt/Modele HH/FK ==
  note: gkm
  note: (Vm-Vk0)
  FKIn : Inport  Port=1  LatchInput=off
  (Vm-Vk0) : Fcn  Expr=(u-Vk)
  Product : Product
  n(Vm) : Subsystem
  n^4 : Fcn  Expr=gk*(u^4)
  FKout : Outport  InitialOutput=0
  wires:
  n(Vm)/1(n) -> n^4/1
  (Vm-Vk0)/1 -> Product/2
  Product/1 -> FKout/1
  n^4/1 -> Product/1
  FKIn/1 -> n(Vm)/1(Vm), (Vm-Vk0)/1

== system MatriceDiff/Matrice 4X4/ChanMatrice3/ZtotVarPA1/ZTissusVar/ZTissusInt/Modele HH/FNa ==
  note: gNa*m^3
  note: m
  note: h
  note: gNam
  note: (Vm-VNa0)
  FNaIn : Inport  Port=1  LatchInput=off
  (Vm-VNa0) : Fcn  Expr=(u-Vna)
  Product : Product
  Product1 : Product
  gna*m^3 : Fcn  Expr=gna*u^3
  h(Vm) : Subsystem
  m(Vm) : Subsystem
  FNaOut : Outport  InitialOutput=0
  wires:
  (Vm-VNa0)/1 -> Product1/2
  gna*m^3/1 -> Product/1
  Product1/1 -> FNaOut/1
  FNaIn/1 -> m(Vm)/1(Vm), h(Vm)/1(Vm), (Vm-VNa0)/1
  m(Vm)/1(n) -> gna*m^3/1
  h(Vm)/1(h) -> Product/2
  Product/1 -> Product1/1

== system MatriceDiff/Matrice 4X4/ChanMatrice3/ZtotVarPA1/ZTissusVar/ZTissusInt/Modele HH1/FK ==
  note: gkm
  note: (Vm-Vk0)
  FKIn : Inport  Port=1  LatchInput=off
  (Vm-Vk0) : Fcn  Expr=(u-Vk)
  Product : Product
  n(Vm) : Subsystem
  n^4 : Fcn  Expr=gk*(u^4)
  FKout : Outport  InitialOutput=0
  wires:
  n(Vm)/1(n) -> n^4/1
  (Vm-Vk0)/1 -> Product/2
  Product/1 -> FKout/1
  n^4/1 -> Product/1
  FKIn/1 -> n(Vm)/1(Vm), (Vm-Vk0)/1

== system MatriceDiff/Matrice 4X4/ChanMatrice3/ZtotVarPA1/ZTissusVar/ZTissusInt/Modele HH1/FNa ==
  note: gNa*m^3
  note: m
  note: h
  note: gNam
  note: (Vm-VNa0)
  FNaIn : Inport  Port=1  LatchInput=off
  (Vm-VNa0) : Fcn  Expr=(u-Vna)
  Product : Product
  Product1 : Product
  gna*m^3 : Fcn  Expr=gna*u^3
  h(Vm) : Subsystem
  m(Vm) : Subsystem
  FNaOut : Outport  InitialOutput=0
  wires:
  (Vm-VNa0)/1 -> Product1/2
  gna*m^3/1 -> Product/1
  Product1/1 -> FNaOut/1
  FNaIn/1 -> m(Vm)/1(Vm), h(Vm)/1(Vm), (Vm-VNa0)/1
  m(Vm)/1(n) -> gna*m^3/1
  h(Vm)/1(h) -> Product/2
  Product/1 -> Product1/1

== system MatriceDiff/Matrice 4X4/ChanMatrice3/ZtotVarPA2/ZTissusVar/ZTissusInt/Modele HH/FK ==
  note: gkm
  note: (Vm-Vk0)
  FKIn : Inport  Port=1  LatchInput=off
  (Vm-Vk0) : Fcn  Expr=(u-Vk)
  Product : Product
  n(Vm) : Subsystem
  n^4 : Fcn  Expr=gk*(u^4)
  FKout : Outport  InitialOutput=0
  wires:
  n(Vm)/1(n) -> n^4/1
  (Vm-Vk0)/1 -> Product/2
  Product/1 -> FKout/1
  n^4/1 -> Product/1
  FKIn/1 -> n(Vm)/1(Vm), (Vm-Vk0)/1

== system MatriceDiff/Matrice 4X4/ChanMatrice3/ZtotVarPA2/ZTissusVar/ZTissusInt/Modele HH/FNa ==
  note: gNa*m^3
  note: m
  note: h
  note: gNam
  note: (Vm-VNa0)
  FNaIn : Inport  Port=1  LatchInput=off
  (Vm-VNa0) : Fcn  Expr=(u-Vna)
  Product : Product
  Product1 : Product
  gna*m^3 : Fcn  Expr=gna*u^3
  h(Vm) : Subsystem
  m(Vm) : Subsystem
  FNaOut : Outport  InitialOutput=0
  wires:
  (Vm-VNa0)/1 -> Product1/2
  gna*m^3/1 -> Product/1
  Product1/1 -> FNaOut/1
  FNaIn/1 -> m(Vm)/1(Vm), h(Vm)/1(Vm), (Vm-VNa0)/1
  m(Vm)/1(n) -> gna*m^3/1
  h(Vm)/1(h) -> Product/2
  Product/1 -> Product1/1

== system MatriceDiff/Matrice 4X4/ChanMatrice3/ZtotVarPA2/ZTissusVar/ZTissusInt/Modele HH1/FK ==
  note: gkm
  note: (Vm-Vk0)
  FKIn : Inport  Port=1  LatchInput=off
  (Vm-Vk0) : Fcn  Expr=(u-Vk)
  Product : Product
  n(Vm) : Subsystem
  n^4 : Fcn  Expr=gk*(u^4)
  FKout : Outport  InitialOutput=0
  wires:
  n(Vm)/1(n) -> n^4/1
  (Vm-Vk0)/1 -> Product/2
  Product/1 -> FKout/1
  n^4/1 -> Product/1
  FKIn/1 -> n(Vm)/1(Vm), (Vm-Vk0)/1

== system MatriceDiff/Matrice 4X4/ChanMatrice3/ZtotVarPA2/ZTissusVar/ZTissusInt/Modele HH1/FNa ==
  note: gNa*m^3
  note: m
  note: h
  note: gNam
  note: (Vm-VNa0)
  FNaIn : Inport  Port=1  LatchInput=off
  (Vm-VNa0) : Fcn  Expr=(u-Vna)
  Product : Product
  Product1 : Product
  gna*m^3 : Fcn  Expr=gna*u^3
  h(Vm) : Subsystem
  m(Vm) : Subsystem
  FNaOut : Outport  InitialOutput=0
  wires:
  (Vm-VNa0)/1 -> Product1/2
  gna*m^3/1 -> Product/1
  Product1/1 -> FNaOut/1
  FNaIn/1 -> m(Vm)/1(Vm), h(Vm)/1(Vm), (Vm-VNa0)/1
  m(Vm)/1(n) -> gna*m^3/1
  h(Vm)/1(h) -> Product/2
  Product/1 -> Product1/1

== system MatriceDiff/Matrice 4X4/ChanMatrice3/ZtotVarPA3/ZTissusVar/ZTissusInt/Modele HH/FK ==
  note: gkm
  note: (Vm-Vk0)
  FKIn : Inport  Port=1  LatchInput=off
  (Vm-Vk0) : Fcn  Expr=(u-Vk)
  Product : Product
  n(Vm) : Subsystem
  n^4 : Fcn  Expr=gk*(u^4)
  FKout : Outport  InitialOutput=0
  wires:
  n(Vm)/1(n) -> n^4/1
  (Vm-Vk0)/1 -> Product/2
  Product/1 -> FKout/1
  n^4/1 -> Product/1
  FKIn/1 -> n(Vm)/1(Vm), (Vm-Vk0)/1

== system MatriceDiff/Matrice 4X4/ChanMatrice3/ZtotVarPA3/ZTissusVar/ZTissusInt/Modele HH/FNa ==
  note: gNa*m^3
  note: m
  note: h
  note: gNam
  note: (Vm-VNa0)
  FNaIn : Inport  Port=1  LatchInput=off
  (Vm-VNa0) : Fcn  Expr=(u-Vna)
  Product : Product
  Product1 : Product
  gna*m^3 : Fcn  Expr=gna*u^3
  h(Vm) : Subsystem
  m(Vm) : Subsystem
  FNaOut : Outport  InitialOutput=0
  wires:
  (Vm-VNa0)/1 -> Product1/2
  gna*m^3/1 -> Product/1
  Product1/1 -> FNaOut/1
  FNaIn/1 -> m(Vm)/1(Vm), h(Vm)/1(Vm), (Vm-VNa0)/1
  m(Vm)/1(n) -> gna*m^3/1
  h(Vm)/1(h) -> Product/2
  Product/1 -> Product1/1

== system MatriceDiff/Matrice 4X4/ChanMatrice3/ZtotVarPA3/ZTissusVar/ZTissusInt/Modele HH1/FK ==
  note: gkm
  note: (Vm-Vk0)
  FKIn : Inport  Port=1  LatchInput=off
  (Vm-Vk0) : Fcn  Expr=(u-Vk)
  Product : Product
  n(Vm) : Subsystem
  n^4 : Fcn  Expr=gk*(u^4)
  FKout : Outport  InitialOutput=0
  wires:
  n(Vm)/1(n) -> n^4/1
  (Vm-Vk0)/1 -> Product/2
  Product/1 -> FKout/1
  n^4/1 -> Product/1
  FKIn/1 -> n(Vm)/1(Vm), (Vm-Vk0)/1

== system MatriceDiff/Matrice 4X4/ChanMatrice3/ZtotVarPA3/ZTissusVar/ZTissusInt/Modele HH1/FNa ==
  note: gNa*m^3
  note: m
  note: h
  note: gNam
  note: (Vm-VNa0)
  FNaIn : Inport  Port=1  LatchInput=off
  (Vm-VNa0) : Fcn  Expr=(u-Vna)
  Product : Product
  Product1 : Product
  gna*m^3 : Fcn  Expr=gna*u^3
  h(Vm) : Subsystem
  m(Vm) : Subsystem
  FNaOut : Outport  InitialOutput=0
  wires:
  (Vm-VNa0)/1 -> Product1/2
  gna*m^3/1 -> Product/1
  Product1/1 -> FNaOut/1
  FNaIn/1 -> m(Vm)/1(Vm), h(Vm)/1(Vm), (Vm-VNa0)/1
  m(Vm)/1(n) -> gna*m^3/1
  h(Vm)/1(h) -> Product/2
  Product/1 -> Product1/1

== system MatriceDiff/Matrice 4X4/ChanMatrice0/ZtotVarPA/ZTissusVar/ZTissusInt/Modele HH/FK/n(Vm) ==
  note: V
  note: alpha_*(1-n)
  note: beta_n*n
  note: n
  note: n
  Vm : Inport  Port=1  LatchInput=off
  (1-n) : Fcn  Expr=1-u
  Integrator1 : Integrator  InitialCondition=n0
  Product : Product
  Product1 : Product
  Sum1 : Sum  Inputs=+-
  V : Fcn  Expr=u-Vr
  alpha_n : Fcn  Expr=(0.01*(10-u))/(exp((10-u)/10)-1)
  beta_n : Fcn  Expr=0.125*exp(-u/80)
  n : Outport  InitialOutput=0
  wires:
  V/1 -> alpha_n/1, beta_n/1
  alpha_n/1 -> Product/2
  (1-n)/1 -> Product/1
  beta_n/1 -> Product1/1
  Product/1 -> Sum1/1
  Product1/1 -> Sum1/2
  Sum1/1 -> Integrator1/1
  Integrator1/1 -> (1-n)/1, Product1/2, n/1
  Vm/1 -> V/1

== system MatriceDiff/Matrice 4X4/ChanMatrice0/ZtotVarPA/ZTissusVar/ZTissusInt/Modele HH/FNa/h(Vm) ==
  note: h
  note: h
  note: beta_h*h
  note: alpha_h*(1-h)
  note: V
  Vm : Inport  Port=1  LatchInput=off
  (1-h) : Fcn  Expr=1-u
  Integrator1 : Integrator  InitialCondition=h0
  Product : Product
  Product1 : Product
  Sum1 : Sum  Inputs=+-
  V : Fcn  Expr=u-Vr
  alpha_h : Fcn  Expr=0.07*exp(-u/20)
  beta_h : Fcn  Expr=1/(exp((30-u)/10)+1)
  h : Outport  InitialOutput=0
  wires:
  Vm/1 -> V/1
  Integrator1/1 -> h/1, Product1/2, (1-h)/1
  Sum1/1 -> Integrator1/1
  Product1/1 -> Sum1/2
  Product/1 -> Sum1/1
  beta_h/1 -> Product1/1
  (1-h)/1 -> Product/1
  alpha_h/1 -> Product/2
  V/1 -> beta_h/1, alpha_h/1

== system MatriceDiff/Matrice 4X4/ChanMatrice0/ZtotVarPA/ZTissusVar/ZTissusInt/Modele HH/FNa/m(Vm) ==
  note: m
  note: m
  note: beta_m*m
  note: alpha_m*(1-m)
  note: V
  Vm : Inport  Port=1  LatchInput=off
  (1-m) : Fcn  Expr=1-u
  Integrator1 : Integrator  InitialCondition=m0
  Product : Product
  Product1 : Product
  Sum1 : Sum  Inputs=+-
  V : Fcn  Expr=u-Vr
  alpha_m : Fcn  Expr=(0.1*(25-u))/(exp((25-u)/10)-1)
  beta_m : Fcn  Expr=4*exp(-u/18)
  n : Outport  InitialOutput=0
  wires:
  Vm/1 -> V/1
  Integrator1/1 -> n/1, Product1/2, (1-m)/1
  Sum1/1 -> Integrator1/1
  Product1/1 -> Sum1/2
  Product/1 -> Sum1/1
  beta_m/1 -> Product1/1
  (1-m)/1 -> Product/1
  alpha_m/1 -> Product/2
  V/1 -> beta_m/1, alpha_m/1

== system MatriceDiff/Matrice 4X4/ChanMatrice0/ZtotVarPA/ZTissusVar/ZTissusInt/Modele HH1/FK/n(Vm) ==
  note: V
  note: alpha_*(1-n)
  note: beta_n*n
  note: n
  note: n
  Vm : Inport  Port=1  LatchInput=off
  (1-n) : Fcn  Expr=1-u
  Integrator1 : Integrator  InitialCondition=n0
  Product : Product
  Product1 : Product
  Sum1 : Sum  Inputs=+-
  V : Fcn  Expr=u-Vr
  alpha_n : Fcn  Expr=(0.01*(10-u))/(exp((10-u)/10)-1)
  beta_n : Fcn  Expr=0.125*exp(-u/80)
  n : Outport  InitialOutput=0
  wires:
  V/1 -> alpha_n/1, beta_n/1
  alpha_n/1 -> Product/2
  (1-n)/1 -> Product/1
  beta_n/1 -> Product1/1
  Product/1 -> Sum1/1
  Product1/1 -> Sum1/2
  Sum1/1 -> Integrator1/1
  Integrator1/1 -> (1-n)/1, Product1/2, n/1
  Vm/1 -> V/1

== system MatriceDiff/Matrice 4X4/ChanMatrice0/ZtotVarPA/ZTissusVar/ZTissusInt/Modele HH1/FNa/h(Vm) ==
  note: h
  note: h
  note: beta_h*h
  note: alpha_h*(1-h)
  note: V
  Vm : Inport  Port=1  LatchInput=off
  (1-h) : Fcn  Expr=1-u
  Integrator1 : Integrator  InitialCondition=h0
  Product : Product
  Product1 : Product
  Sum1 : Sum  Inputs=+-
  V : Fcn  Expr=u-Vr
  alpha_h : Fcn  Expr=0.07*exp(-u/20)
  beta_h : Fcn  Expr=1/(exp((30-u)/10)+1)
  h : Outport  InitialOutput=0
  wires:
  Vm/1 -> V/1
  Integrator1/1 -> h/1, Product1/2, (1-h)/1
  Sum1/1 -> Integrator1/1
  Product1/1 -> Sum1/2
  Product/1 -> Sum1/1
  beta_h/1 -> Product1/1
  (1-h)/1 -> Product/1
  alpha_h/1 -> Product/2
  V/1 -> beta_h/1, alpha_h/1

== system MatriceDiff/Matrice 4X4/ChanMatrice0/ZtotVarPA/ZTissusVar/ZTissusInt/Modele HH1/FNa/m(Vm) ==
  note: m
  note: m
  note: beta_m*m
  note: alpha_m*(1-m)
  note: V
  Vm : Inport  Port=1  LatchInput=off
  (1-m) : Fcn  Expr=1-u
  Integrator1 : Integrator  InitialCondition=m0
  Product : Product
  Product1 : Product
  Sum1 : Sum  Inputs=+-
  V : Fcn  Expr=u-Vr
  alpha_m : Fcn  Expr=(0.1*(25-u))/(exp((25-u)/10)-1)
  beta_m : Fcn  Expr=4*exp(-u/18)
  n : Outport  InitialOutput=0
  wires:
  Vm/1 -> V/1
  Integrator1/1 -> n/1, Product1/2, (1-m)/1
  Sum1/1 -> Integrator1/1
  Product1/1 -> Sum1/2
  Product/1 -> Sum1/1
  beta_m/1 -> Product1/1
  (1-m)/1 -> Product/1
  alpha_m/1 -> Product/2
  V/1 -> beta_m/1, alpha_m/1

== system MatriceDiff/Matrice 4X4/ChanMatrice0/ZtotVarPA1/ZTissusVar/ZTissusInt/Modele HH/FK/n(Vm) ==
  note: V
  note: alpha_*(1-n)
  note: beta_n*n
  note: n
  note: n
  Vm : Inport  Port=1  LatchInput=off
  (1-n) : Fcn  Expr=1-u
  Integrator1 : Integrator  InitialCondition=n0
  Product : Product
  Product1 : Product
  Sum1 : Sum  Inputs=+-
  V : Fcn  Expr=u-Vr
  alpha_n : Fcn  Expr=(0.01*(10-u))/(exp((10-u)/10)-1)
  beta_n : Fcn  Expr=0.125*exp(-u/80)
  n : Outport  InitialOutput=0
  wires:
  V/1 -> alpha_n/1, beta_n/1
  alpha_n/1 -> Product/2
  (1-n)/1 -> Product/1
  beta_n/1 -> Product1/1
  Product/1 -> Sum1/1
  Product1/1 -> Sum1/2
  Sum1/1 -> Integrator1/1
  Integrator1/1 -> (1-n)/1, Product1/2, n/1
  Vm/1 -> V/1

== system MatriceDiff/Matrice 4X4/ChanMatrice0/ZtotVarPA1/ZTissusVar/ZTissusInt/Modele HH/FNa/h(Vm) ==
  note: h
  note: h
  note: beta_h*h
  note: alpha_h*(1-h)
  note: V
  Vm : Inport  Port=1  LatchInput=off
  (1-h) : Fcn  Expr=1-u
  Integrator1 : Integrator  InitialCondition=h0
  Product : Product
  Product1 : Product
  Sum1 : Sum  Inputs=+-
  V : Fcn  Expr=u-Vr
  alpha_h : Fcn  Expr=0.07*exp(-u/20)
  beta_h : Fcn  Expr=1/(exp((30-u)/10)+1)
  h : Outport  InitialOutput=0
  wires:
  Vm/1 -> V/1
  Integrator1/1 -> h/1, Product1/2, (1-h)/1
  Sum1/1 -> Integrator1/1
  Product1/1 -> Sum1/2
  Product/1 -> Sum1/1
  beta_h/1 -> Product1/1
  (1-h)/1 -> Product/1
  alpha_h/1 -> Product/2
  V/1 -> beta_h/1, alpha_h/1

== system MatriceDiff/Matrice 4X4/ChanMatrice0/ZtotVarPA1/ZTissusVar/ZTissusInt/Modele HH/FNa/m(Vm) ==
  note: m
  note: m
  note: beta_m*m
  note: alpha_m*(1-m)
  note: V
  Vm : Inport  Port=1  LatchInput=off
  (1-m) : Fcn  Expr=1-u
  Integrator1 : Integrator  InitialCondition=m0
  Product : Product
  Product1 : Product
  Sum1 : Sum  Inputs=+-
  V : Fcn  Expr=u-Vr
  alpha_m : Fcn  Expr=(0.1*(25-u))/(exp((25-u)/10)-1)
  beta_m : Fcn  Expr=4*exp(-u/18)
  n : Outport  InitialOutput=0
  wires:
  Vm/1 -> V/1
  Integrator1/1 -> n/1, Product1/2, (1-m)/1
  Sum1/1 -> Integrator1/1
  Product1/1 -> Sum1/2
  Product/1 -> Sum1/1
  beta_m/1 -> Product1/1
  (1-m)/1 -> Product/1
  alpha_m/1 -> Product/2
  V/1 -> beta_m/1, alpha_m/1

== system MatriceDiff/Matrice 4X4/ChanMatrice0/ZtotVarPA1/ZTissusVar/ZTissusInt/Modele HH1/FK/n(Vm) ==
  note: V
  note: alpha_*(1-n)
  note: beta_n*n
  note: n
  note: n
  Vm : Inport  Port=1  LatchInput=off
  (1-n) : Fcn  Expr=1-u
  Integrator1 : Integrator  InitialCondition=n0
  Product : Product
  Product1 : Product
  Sum1 : Sum  Inputs=+-
  V : Fcn  Expr=u-Vr
  alpha_n : Fcn  Expr=(0.01*(10-u))/(exp((10-u)/10)-1)
  beta_n : Fcn  Expr=0.125*exp(-u/80)
  n : Outport  InitialOutput=0
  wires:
  V/1 -> alpha_n/1, beta_n/1
  alpha_n/1 -> Product/2
  (1-n)/1 -> Product/1
  beta_n/1 -> Product1/1
  Product/1 -> Sum1/1
  Product1/1 -> Sum1/2
  Sum1/1 -> Integrator1/1
  Integrator1/1 -> (1-n)/1, Product1/2, n/1
  Vm/1 -> V/1

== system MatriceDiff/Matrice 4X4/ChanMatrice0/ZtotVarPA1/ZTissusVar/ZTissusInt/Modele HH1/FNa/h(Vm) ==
  note: h
  note: h
  note: beta_h*h
  note: alpha_h*(1-h)
  note: V
  Vm : Inport  Port=1  LatchInput=off
  (1-h) : Fcn  Expr=1-u
  Integrator1 : Integrator  InitialCondition=h0
  Product : Product
  Product1 : Product
  Sum1 : Sum  Inputs=+-
  V : Fcn  Expr=u-Vr
  alpha_h : Fcn  Expr=0.07*exp(-u/20)
  beta_h : Fcn  Expr=1/(exp((30-u)/10)+1)
  h : Outport  InitialOutput=0
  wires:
  Vm/1 -> V/1
  Integrator1/1 -> h/1, Product1/2, (1-h)/1
  Sum1/1 -> Integrator1/1
  Product1/1 -> Sum1/2
  Product/1 -> Sum1/1
  beta_h/1 -> Product1/1
  (1-h)/1 -> Product/1
  alpha_h/1 -> Product/2
  V/1 -> beta_h/1, alpha_h/1

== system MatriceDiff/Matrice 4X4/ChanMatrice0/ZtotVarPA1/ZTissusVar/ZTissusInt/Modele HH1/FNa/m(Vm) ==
  note: m
  note: m
  note: beta_m*m
  note: alpha_m*(1-m)
  note: V
  Vm : Inport  Port=1  LatchInput=off
  (1-m) : Fcn  Expr=1-u
  Integrator1 : Integrator  InitialCondition=m0
  Product : Product
  Product1 : Product
  Sum1 : Sum  Inputs=+-
  V : Fcn  Expr=u-Vr
  alpha_m : Fcn  Expr=(0.1*(25-u))/(exp((25-u)/10)-1)
  beta_m : Fcn  Expr=4*exp(-u/18)
  n : Outport  InitialOutput=0
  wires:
  Vm/1 -> V/1
  Integrator1/1 -> n/1, Product1/2, (1-m)/1
  Sum1/1 -> Integrator1/1
  Product1/1 -> Sum1/2
  Product/1 -> Sum1/1
  beta_m/1 -> Product1/1
  (1-m)/1 -> Product/1
  alpha_m/1 -> Product/2
  V/1 -> beta_m/1, alpha_m/1

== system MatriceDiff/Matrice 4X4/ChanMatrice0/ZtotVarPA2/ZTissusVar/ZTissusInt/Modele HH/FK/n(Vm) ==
  note: V
  note: alpha_*(1-n)
  note: beta_n*n
  note: n
  note: n
  Vm : Inport  Port=1  LatchInput=off
  (1-n) : Fcn  Expr=1-u
  Integrator1 : Integrator  InitialCondition=n0
  Product : Product
  Product1 : Product
  Sum1 : Sum  Inputs=+-
  V : Fcn  Expr=u-Vr
  alpha_n : Fcn  Expr=(0.01*(10-u))/(exp((10-u)/10)-1)
  beta_n : Fcn  Expr=0.125*exp(-u/80)
  n : Outport  InitialOutput=0
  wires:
  V/1 -> alpha_n/1, beta_n/1
  alpha_n/1 -> Product/2
  (1-n)/1 -> Product/1
  beta_n/1 -> Product1/1
  Product/1 -> Sum1/1
  Product1/1 -> Sum1/2
  Sum1/1 -> Integrator1/1
  Integrator1/1 -> (1-n)/1, Product1/2, n/1
  Vm/1 -> V/1

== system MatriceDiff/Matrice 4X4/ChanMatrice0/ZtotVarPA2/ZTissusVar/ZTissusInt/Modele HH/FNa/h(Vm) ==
  note: h
  note: h
  note: beta_h*h
  note: alpha_h*(1-h)
  note: V
  Vm : Inport  Port=1  LatchInput=off
  (1-h) : Fcn  Expr=1-u
  Integrator1 : Integrator  InitialCondition=h0
  Product : Product
  Product1 : Product
  Sum1 : Sum  Inputs=+-
  V : Fcn  Expr=u-Vr
  alpha_h : Fcn  Expr=0.07*exp(-u/20)
  beta_h : Fcn  Expr=1/(exp((30-u)/10)+1)
  h : Outport  InitialOutput=0
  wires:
  Vm/1 -> V/1
  Integrator1/1 -> h/1, Product1/2, (1-h)/1
  Sum1/1 -> Integrator1/1
  Product1/1 -> Sum1/2
  Product/1 -> Sum1/1
  beta_h/1 -> Product1/1
  (1-h)/1 -> Product/1
  alpha_h/1 -> Product/2
  V/1 -> beta_h/1, alpha_h/1

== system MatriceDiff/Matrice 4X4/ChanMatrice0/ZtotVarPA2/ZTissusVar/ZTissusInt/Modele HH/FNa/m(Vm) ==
  note: m
  note: m
  note: beta_m*m
  note: alpha_m*(1-m)
  note: V
  Vm : Inport  Port=1  LatchInput=off
  (1-m) : Fcn  Expr=1-u
  Integrator1 : Integrator  InitialCondition=m0
  Product : Product
  Product1 : Product
  Sum1 : Sum  Inputs=+-
  V : Fcn  Expr=u-Vr
  alpha_m : Fcn  Expr=(0.1*(25-u))/(exp((25-u)/10)-1)
  beta_m : Fcn  Expr=4*exp(-u/18)
  n : Outport  InitialOutput=0
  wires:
  Vm/1 -> V/1
  Integrator1/1 -> n/1, Product1/2, (1-m)/1
  Sum1/1 -> Integrator1/1
  Product1/1 -> Sum1/2
  Product/1 -> Sum1/1
  beta_m/1 -> Product1/1
  (1-m)/1 -> Product/1
  alpha_m/1 -> Product/2
  V/1 -> beta_m/1, alpha_m/1
